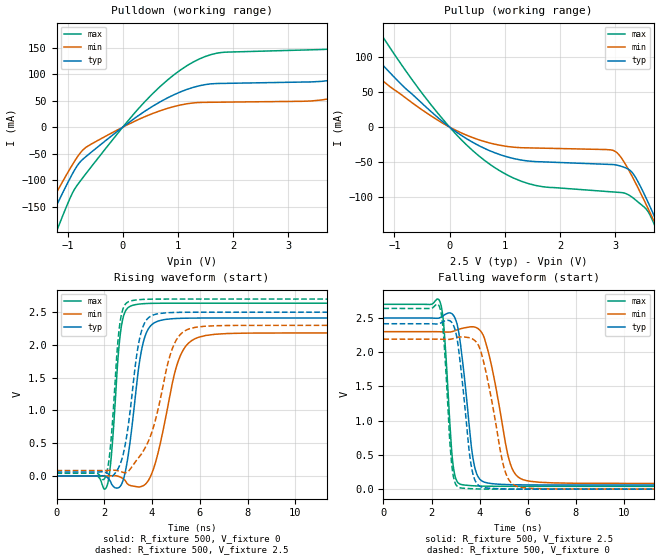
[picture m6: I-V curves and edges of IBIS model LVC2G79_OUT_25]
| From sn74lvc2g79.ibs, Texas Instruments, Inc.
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[Model]   LVC2G79_OUT_25
Model_type  Output
Vref =   0
Rref =   500
Cref =   30p
Vmeas =   1.25
| variable   typ   min   max
C_comp   9.80pF   6.16pF   14.72pF
| C_pullup   9.65pF   6.16pF   11.31pF
| C_pulldown   9.95pF   6.65pF   14.72pF
[Temperature Range]   40   100   -40
| Ambient temperature   25   85   -40
[Voltage range]   2.5   2.3   2.7
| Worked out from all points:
|   slope of the pulldown table from 0 to 0.375 V, typ, clamps not added: 13.3 ohm
|   slope of the pullup table from 0 to 0.375 V, typ, clamps not added: 19 ohm
|   rising waveform, R_fixture 500, V_fixture 0: 20-80 % time 499ps typ, 783ps min, 308ps max; typ from 0 V to 2.41 V
|   falling waveform, R_fixture 500, V_fixture 2.5: 20-80 % time 442ps typ, 696ps min, 278ps max; typ from 2.5 V to 0.061 V
|   rising waveform, R_fixture 500, V_fixture 2.5: 20-80 % time 522ps typ, 927ps min, 312ps max; typ from 0.061 V to 2.5 V
|   falling waveform, R_fixture 500, V_fixture 0: 20-80 % time 428ps typ, 693ps min, 269ps max; typ from 2.42 V to 0 V
[Pulldown]
| LVC2G79_OUT_25
|   Voltage   I(typ)   I(min)   I(max)
-5.5V     -1.06A     -941.4mA   -1.275A
-1.52V    -217.1mA   -184.1mA   -281.2mA
-1.26V    -160.6mA   -134.6mA   -212.3mA
-665mV    -55.38mA   -37.96mA   -87.52mA
385mV     28.96mA    19.04mA    46.35mA
1.275V    74.94mA    45.66mA    122.7mA
3.82V     89.63mA    55.12mA    148.2mA
5.34V     157.4mA    105.8mA    232mA
5.91V     188.7mA    52.55mA    283.4mA
6.525V    93.54mA    53.06mA    299.5mA
7.555V    94.08mA    54.03mA    161.4mA
11V       99.63mA    57.49mA    169.6mA
[Pullup]
| LVC2G79_OUT_25
|   Voltage   I(typ)   I(min)   I(max)
-5.5V     533.4mA    418.6mA    746.4mA
-2.335V   192.2mA    147mA      274.9mA
-1.875V   147.9mA    112.2mA    212.9mA
-1.315V   97.38mA    72.9mA     141.5mA
-225mV    14.47mA    10.42mA    20.98mA
735mV     -33.88mA   -22.76mA   -53.28mA
1.56V     -49.18mA   -29.79mA   -83.17mA
2.98V     -53.48mA   -33.7mA    -92.52mA
3.325V    -66.27mA   -72.72mA   -100.9mA
3.755V    -135mA     -142.5mA   -147.1mA
3.835V    -149.5mA   -156.2mA   -162.8mA
11V       -1.609A    -1.492A    -1.841A
[Ramp]
| LVC2G79_OUT_25
| variable   typ   min   max
dV/dt_r   1.56/5.40E-10   1.41/8.45E-10   1.70/3.32E-10
dV/dt_f   1.51/4.65E-10   1.37/7.25E-10   1.64/2.88E-10
R_load = 500
[Rising Waveform]
| LVC2G79_OUT_25
R_fixture =   500
C_fixture =   0
L_fixture =   0
V_fixture =   0
V_fixture_min = 0
V_fixture_max = 0
|   Time   V(typ)   V(min)   V(max)
0s        125.3pV    6.247nV    2.314nV
2.095ns   -14.38mV   772.8uV    -168.8mV
2.29ns    -108.7mV   4.267mV    287.7mV
2.695ns   -143.1mV   -20.26mV   2.236V
3.175ns   804.3mV    -151.5mV   2.603V
3.515ns   1.832V     -163.3mV   2.626V
3.855ns   2.251V     -62.22mV   2.633V
5.095ns   2.405V     1.753V     2.637V
5.935ns   2.41V      2.116V     2.637V
22ns      2.411V     2.183V     2.637V
[Falling Waveform]
| LVC2G79_OUT_25
R_fixture =   500
C_fixture =   0
L_fixture =   0
V_fixture =   2.5
V_fixture_min = 2.3
V_fixture_max = 2.7
|   Time   V(typ)   V(min)   V(max)
0s        2.5V       2.3V       2.7V
2.34ns    2.503V     2.299V     2.747V
2.5ns     2.537V     2.297V     2.437V
2.88ns    2.552V     2.304V     403.6mV
3.2ns     2.13V      2.342V     71.33mV
3.74ns    420.3mV    2.371V     49.27mV
4.21ns    101.1mV    2.191V     43.94mV
5.225ns   66.22mV    431.2mV    41.77mV
5.82ns    62.89mV    137.3mV    41.6mV
22ns      60.96mV    83.68mV    41.48mV
[Rising Waveform]
| LVC2G79_OUT_25
R_fixture =   500
C_fixture =   0
L_fixture =   0
V_fixture =   2.5
V_fixture_min = 2.3
V_fixture_max = 2.7
|   Time   V(typ)   V(min)   V(max)
0s        60.91mV    83.6mV     41.45mV
2.04ns    57.77mV    83.96mV    -18.37mV
2.26ns    7.964mV    87.21mV    459mV
2.655ns   173mV      72.54mV    2.331V
3.08ns    987.7mV    102.9mV    2.669V
3.4ns     1.945V     263.7mV    2.689V
3.715ns   2.353V     434.2mV    2.696V
4.85ns    2.495V     1.945V     2.7V
5.585ns   2.499V     2.249V     2.7V
22ns      2.5V       2.3V       2.7V
[Falling Waveform]
| LVC2G79_OUT_25
R_fixture =   500
C_fixture =   0
L_fixture =   0
V_fixture =   0
V_fixture_min = 0
V_fixture_max = 0
|   Time   V(typ)   V(min)   V(max)
0s        2.416V     2.191V     2.64V
2.32ns    2.418V     2.191V     2.674V
2.5ns     2.449V     2.188V     2.256V
2.845ns   2.434V     2.193V     348.5mV
3.125ns   2.047V     2.22V      26.54mV
3.65ns    346.9mV    2.203V     6.729mV
4.1ns     30.27mV    1.951V     2.172mV
5.005ns   4.105mV    325.5mV    337.2uV
5.58ns    1.445mV    37.97mV    150uV
22ns      46.01uV    68.3uV     32.74uV
